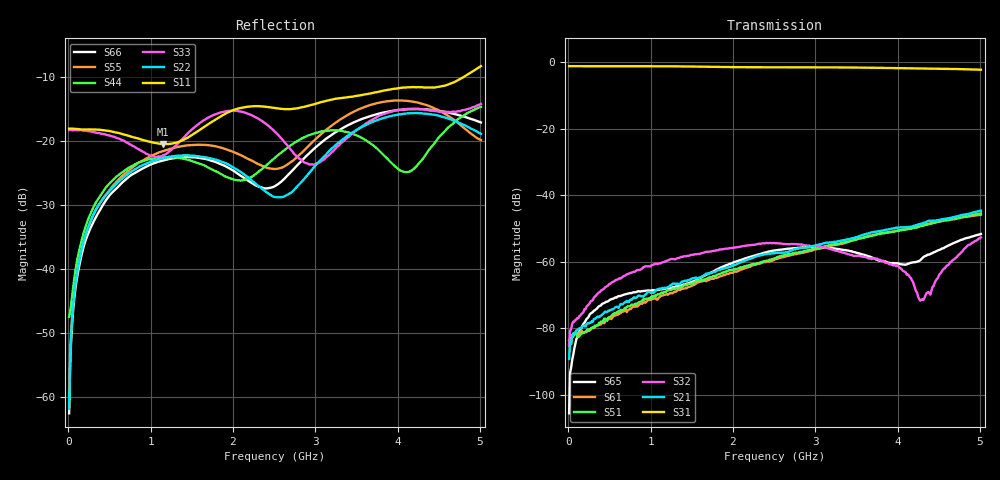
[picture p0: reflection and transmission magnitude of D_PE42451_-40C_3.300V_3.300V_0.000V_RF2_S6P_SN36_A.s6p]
! Device ID: PE42451
! Serial: 36
! Insertion: A
! Temp: -40C
! VDD: 3.300
! Control_Hi: 100.000
! Control_Lo: 0.000
! Logic State: RF2
! Port 1: RFC
! Port 2: RF1
! Port 3: RF2
! Port 4: RF3
! Port 5: RF4
! Port 6: RF5
! V1 = 0.00
! V2 = 3.30
! V3 = 0.00
! V4 = 0.00
! IDD: 1.611260e-05
#  Hz  S  RI  R  50
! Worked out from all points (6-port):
!   401 points, 10 MHz to 5.01 GHz, reference 50 ohm
!   strongest paths, dB at 10 MHz, 1.26 GHz, 2.51 GHz, 3.76 GHz, 5.01 GHz:
!     S31: -1.2, -1.3, -1.6, -1.7, -2.3
!     S21: -89.2, -66.8, -57.4, -50.8, -44.7
!     S32: -85.1, -59.1, -54.4, -59.2, -52.6
!     S51: -84.8, -68.3, -58.9, -51.7, -45.5
!     S61: -83.6, -69.5, -59.2, -51.6, -45.9
!     S65: -105.5, -67.7, -56.6, -59.5, -51.6
!   lowest |S11| = -20.5 dB at 1.147 GHz (marker M1), VSWR 1.21, Z = 56.7 - j7.54 ohm
!   |S11| at or under -10 dB: start of sweep to 4.806 GHz
